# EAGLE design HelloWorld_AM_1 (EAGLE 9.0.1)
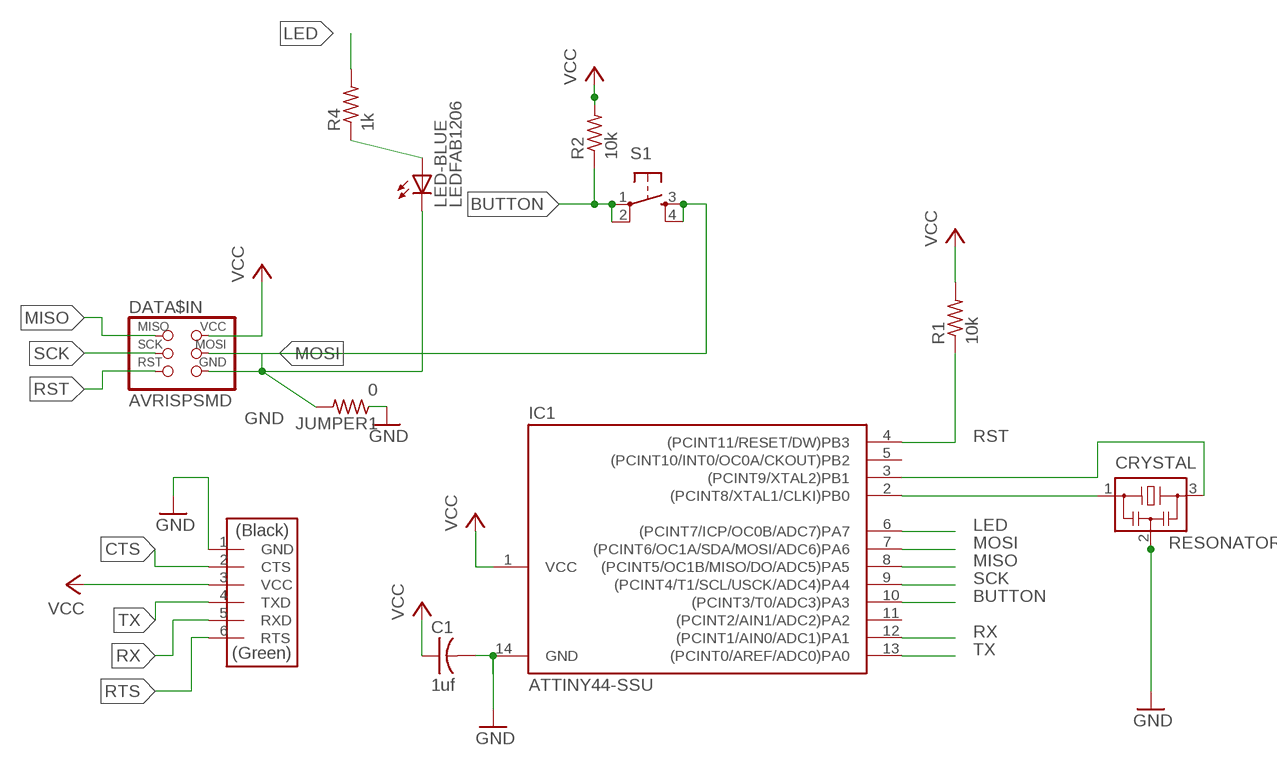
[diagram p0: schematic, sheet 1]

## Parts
C1  1uf  CAP-US1206FAB  [C1206FAB]
CRYSTAL  RESONATOR  [EFOBM]
DATA$IN  AVRISPSMD  [2X03SMD]
DATA$OUT  FTDI-SMD-HEADER  [1X06SMD]
IC1  ATTINY44-SSU  [SOIC14]
JUMPER1  0  RES-US1206FAB  [R1206FAB]
LED-BLUE  LEDFAB1206  [LED1206FAB]
R1  10k  RES-US1206FAB  [R1206FAB]
R2  10k  RES-US1206FAB  [R1206FAB]
R4  1k  RES-US1206FAB  [R1206FAB]
S1  6MM_SWITCH6MM_SWITCH  [6MM_SWITCH]

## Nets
BUTTON: IC1.10((PCINT3/T0/ADC3)PA3) R2.1 S1.1(P) S1.2(P1)
CTS: DATA$OUT.2(CTS)
GND: C1.2 CRYSTAL.2 DATA$IN.6(GND) DATA$OUT.1(GND) IC1.14(GND) JUMPER1.1 JUMPER1.2 LED-BLUE.2(C) S1.3(S) S1.4(S1)
LED: IC1.6((PCINT7/ICP/OC0B/ADC7)PA7) R4.2
MISO: DATA$IN.1(MISO) IC1.8((PCINT5/OC1B/MISO/DO/ADC5)PA5)
MOSI: DATA$IN.4(MOSI) IC1.7((PCINT6/OC1A/SDA/MOSI/ADC6)PA6)
N$1: CRYSTAL.1 IC1.2((PCINT8/XTAL1/CLKI)PB0)
N$3: LED-BLUE.1(A) R4.1
N$7: CRYSTAL.3 IC1.3((PCINT9/XTAL2)PB1)
RST: DATA$IN.5(RST) IC1.4((PCINT11/RESET/DW)PB3) R1.1
RTS: DATA$OUT.6(RTS)
RX: DATA$OUT.5(RXD) IC1.12((PCINT1/AIN0/ADC1)PA1)
SCK: DATA$IN.3(SCK) IC1.9((PCINT4/T1/SCL/USCK/ADC4)PA4)
TX: DATA$OUT.4(TXD) IC1.13((PCINT0/AREF/ADC0)PA0)
VCC: C1.1 DATA$IN.2(VCC) DATA$OUT.3(VCC) IC1.1(VCC) R1.2 R2.2
Unconnected: IC1.5((PCINT10/INT0/OC0A/CKOUT)PB2) IC1.11((PCINT2/AIN1/ADC2)PA2)

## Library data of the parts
C1 = fab:CAP-US
CRYSTAL = fab:RESONATOR
DATA$IN = fab:AVRISP
DATA$OUT = fab:FTDI-SMD-HEADER
IC1 = fab:ATTINY44
JUMPER1 R1 R2 R4 = fab:RES-US: Resistor (US Symbol)
LED-BLUE = fab:LED: LED
S1 = fab:6MM_SWITCH: OMRON SWITCH

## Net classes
0 default: width 0.254 mm, drill 0.508 mm, clearance 0.305 mm

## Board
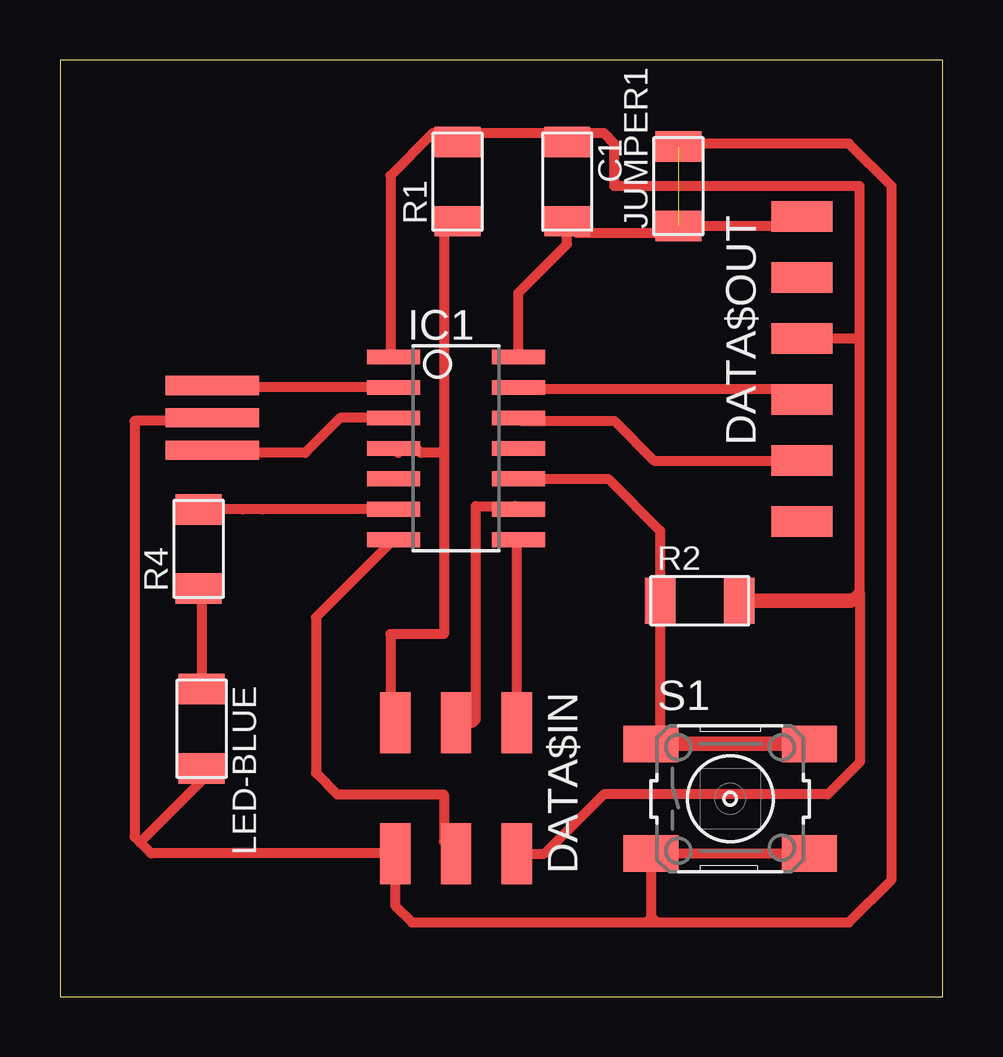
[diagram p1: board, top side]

Size 36.81 x 39.04 mm. Coordinates in mm from the lower left corner, seen from the top.
Outline: 0,0 36.81,0 36.81,39.04 0,39.04 0,0
Copper layers (1*16): Top 0.035mm / dielectric 1.5mm / Bottom 0.035mm
Design rules "default *": minimum track width 16mil, minimum drill 0.35mm, track to track 16mil, track to pad 16mil, pad to pad 16mil, via to via 16mil, smd to smd 16mil, copper to edge 40mil, drill to drill 6mil, minimum pad ring 10mil, minimum via ring 8mil, stop-mask expansion 4mil, vias tented up to drill 0mil, thermal gap 10mil

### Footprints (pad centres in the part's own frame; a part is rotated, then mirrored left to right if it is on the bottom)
C1206FAB = smd 1.27 x 1.905: 1 -1.651,0; 2 1.651,0
EFOBM = smd 0.8 x 3.9: 1 -1.35,0; 2 0,0; 3 1.35,0
2X03SMD = smd 2.54 x 1.27: 1 -2.54,2.54; 2 2.92,2.54; 3 -2.54,0; 4 2.92,0; 5 -2.54,-2.54; 6 2.92,-2.54
1X06SMD = smd 2.54 x 1.27: 1 0,6.35; 2 0,3.81; 3 0,1.27; 4 0,-1.27; 5 0,-3.81; 6 0,-6.35
SOIC14 = smd 0.61 x 2.21: 1 -3.81,-2.603; 2 -2.54,-2.603; 3 -1.27,-2.603; 4 0,-2.603; 5 1.27,-2.603; 6 2.54,-2.603; 7 3.81,-2.603; 8 3.81,2.603; 9 2.54,2.603; 10 1.27,2.603; 11 0,2.603; 12 -1.27,2.603; 13 -2.54,2.603; 14 -3.81,2.603
R1206FAB = smd 1.27 x 1.905: 1 -1.651,0; 2 1.651,0
LED1206FAB = smd 1.27 x 1.905: 1 -1.651,0; 2 1.651,0
6MM_SWITCH = smd 2.286 x 1.524: 1 -3.302,2.286; 2 3.302,2.286; 3 -3.302,-2.286; 4 3.302,-2.286

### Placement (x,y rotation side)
C1  21.15,33.97 270 top
CRYSTAL  6.35,24.13 270 top
DATA$IN  16.51,8.89 270 top
DATA$OUT  30.92,26.16 0 top
IC1  16.51,22.86 270 top
JUMPER1  25.78,33.78 90 top
LED-BLUE  5.91,11.18 270 top
R1  16.57,33.97 90 top
R2  26.67,16.51 0 top
R4  5.78,18.67 90 top
S1  27.94,8.26 0 top

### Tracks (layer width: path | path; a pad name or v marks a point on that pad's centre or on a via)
BUTTON
  Top 0.406: IC1.10 22.86,21.59 25.02,19.43 R2.1 25.02,10.92 S1.1
  Top 0.61: S1.1 S1.2
GND  (1 unrouted)
  Top 0.406: 31.43,32.58 31.56,32.45 31.11,32.45 | 31.11,32.45 30.99,32.45 DATA$OUT.1 | 31.11,32.45 30.8,32.13 JUMPER1.1 25.47,31.82 21.56,31.82 C1.2 21.14,31.37 19.11,29.34 IC1.14 | 13.97,5.14 DATA$IN.6 | DATA$IN.6 13.97,3.81 14.67,3.11 24.45,3.11 | 24.45,3.11 24.89,3.11 | 24.89,3.11 32.89,3.11 34.67,4.89 34.67,33.78 32.89,35.56 25.91,35.56 JUMPER1.2 | 24.64,3.3 24.45,3.11 | S1.4 S1.3 24.64,3.37 24.89,3.11 | DATA$IN.6 | CRYSTAL.2 6.22,24 3.11,24 3.11,6.67 3.33,6.45 | 3.33,6.45 3.78,6 | 3.78,6 3.81,5.97 | LED-BLUE.2 5.91,9.02 3.33,6.45 | 3.78,6 13.94,6 DATA$IN.6
LED
  Top 0.406: IC1.6 8.45,20.32 7.62,20.32 R4.2
MISO
  Top 0.406: 19.11,11.49 DATA$IN.1 19.05,19.05 IC1.8
MOSI
  Top 0.406: IC1.7 10.67,15.81 10.67,9.34 11.56,8.45 16,8.45 16,6.48 DATA$IN.4
N$1
  Top 0.406: IC1.2 6.43,25.4 CRYSTAL.1
N$3
  Top 0.406: R4.1 5.91,16.89 LED-BLUE.1
N$7
  Top 0.406: IC1.3 11.68,24.13 10.22,22.67 6.46,22.67 CRYSTAL.3
RST
  Top 0.406: 14.1,22.67 IC1.4 14.86,22.86 15.05,22.67 16,22.67 | R1.1 16,31.75 16,22.67 | 16,22.67 16,15.11 13.78,15.11 13.78,11.62 DATA$IN.5
RX
  Top 0.406: IC1.12 19.24,24 23.11,24 24.77,22.35 DATA$OUT.5
SCK
  Top 0.406: DATA$IN.3 17.21,11.43 17.34,11.56 17.34,12.89 17.34,20.45 18.99,20.45 IC1.9
TX
  Top 0.406: IC1.13 19.18,25.34 31.11,25.34 31.11,25.08 DATA$OUT.4
VCC
  Top 0.406: DATA$IN.2 20.19,5.97 22.67,8.45 32,8.45 33.34,9.78 33.34,16.89 | 33.34,16.89 33.34,27.56 | 33.34,27.56 33.34,33.78 23.11,33.78 23.11,35.56 22.67,36.01 20.77,36.01 | IC1.1 13.78,26.8 13.78,34.23 15.56,36.01 16.45,36.01 | 32.96,16.51 33.34,16.89 | 16.45,36.01 20.45,36.01 20.77,36.01 | 33.34,27.56 33.21,27.43 DATA$OUT.3 | R1.2 16.57,35.88 16.45,36.01 | C1.1 20.77,36.01
  Top 0.61: R2.2 32.96,16.51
